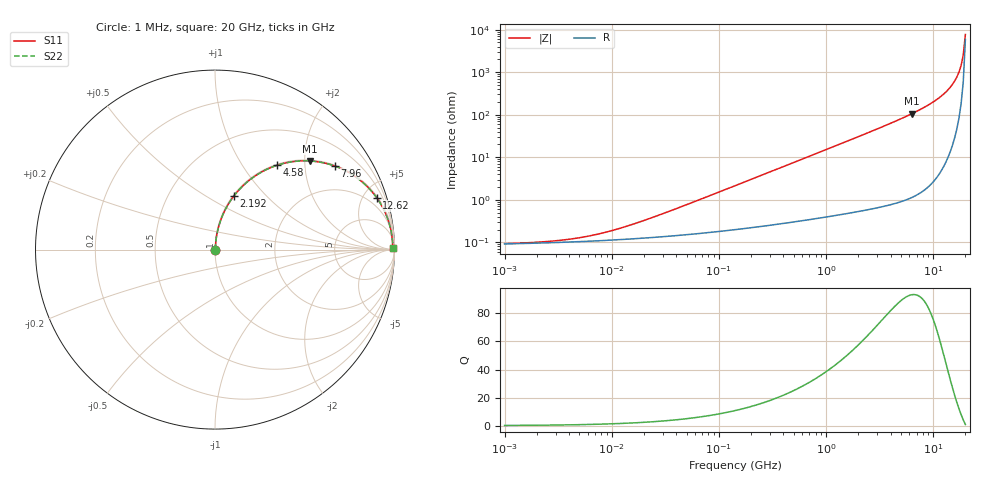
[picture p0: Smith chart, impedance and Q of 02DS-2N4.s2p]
# MHz S MA R 50
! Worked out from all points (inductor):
!   216 points, 1 MHz to 20 GHz, reference 50 ohm
!   read as one part in series: L = 2.4 nH near 26.32 MHz
!   highest Q = 93.2 at 6.323 GHz (marker M1), where L = 2.66 nH
!   S11 on the Smith chart (normalised r, x): 1 MHz: 1.00, +0.00; 2.192 GHz: 1.01, +0.67; 4.58 GHz: 1.02, +1.46; 7.96 GHz: 1.03, +2.84; 12.62 GHz: 1.12, +6.22; 20 GHz: open
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1  0.0009294 9.3  0.9991 -0.0  0.9991 -0.0  0.0009294 9.3
2.63088  0.001055 22.0  0.999 -0.0  0.999 -0.0  0.001055 22.0
5.25016  0.001309 37.1  0.999 -0.0  0.999 -0.0  0.001309 37.1
10.9711  0.002009 55.2  0.9989 -0.1  0.9989 -0.1  0.002009 55.2
27.5642  0.00436 72.0  0.9987 -0.2  0.9987 -0.2  0.00436 72.0
144.716  0.02187 83.5  0.9978 -1.2  0.9978 -1.2  0.02187 83.5
759.783  0.1136 81.7  0.99 -6.5  0.99 -6.5  0.1136 81.7
1382.78  0.2042 77.0  0.9746 -11.8  0.9746 -11.8  0.2042 77.0
2191.8  0.3156 70.7  0.9437 -18.4  0.9437 -18.4  0.3156 70.7
3025.75  0.4207 64.3  0.9014 -24.9  0.9014 -24.9  0.4207 64.3
3988.98  0.5276 57.5  0.8431 -31.8  0.8431 -31.8  0.5276 57.5
4580.12  0.5853 53.5  0.8041 -35.8  0.8041 -35.8  0.5853 53.5
6322.81  0.7224 43.1  0.6838 -46.2  0.6838 -46.2  0.7224 43.1
7960.39  0.8133 34.9  0.5729 -54.4  0.5729 -54.4  0.8133 34.9
10022.1  0.8899 26.4  0.4446 -62.8  0.4446 -62.8  0.8899 26.4
12617.8  0.9465 17.7  0.3044 -71.1  0.3044 -71.1  0.9465 17.7
15170.5  0.9754 10.8  0.1873 -77.1  0.1873 -77.1  0.9754 10.8
16634.5  0.9841 7.3  0.1279 -79.2  0.1279 -79.2  0.9841 7.3
17418.7  0.9871 5.6  0.09822 -79.6  0.09822 -79.6  0.9871 5.6
18239.8  0.9891 3.9  0.06857 -78.9  0.06857 -78.9  0.9891 3.9
19099.6  0.9901 2.2  0.03923 -74.3  0.03923 -74.3  0.9901 2.2
20000  0.9902 0.5  0.01283 -39.8  0.01283 -39.8  0.9902 0.5
